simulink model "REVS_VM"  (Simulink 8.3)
settings: Solver=ode3  StartTime=REVS.sim_start_time_secs  StopTime=Inf  FixedStep=REVS.sim_step_time_secs  MaxStep=REVS.sim_step_time_secs
StopFcn:
  | postproc_datalog;
  | postproc_audit;
  | postproc_result;
model workspace (MATLAB code in the model file):
  other statements: REVS_setup_variants
libraries: vehicle_lib x2, ambient_lib x1, driver_lib x1, accessory_lib x1, electric_lib x1, controls_lib x1, engine_lib x1, transmission_lib x1, simulink x1

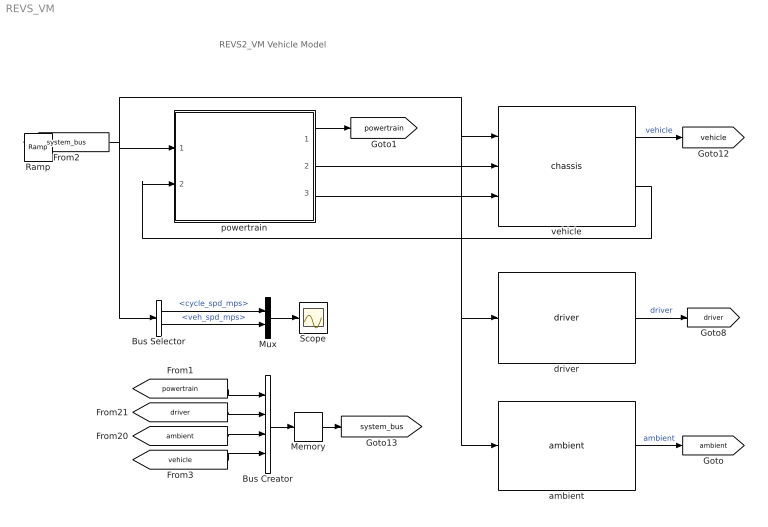
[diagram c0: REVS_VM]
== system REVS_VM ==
  note: REVS2_VM Vehicle Model
  Bus Creator : BusCreator
  Bus Selector : BusSelector  OutputSignals=driver.cycle_spd_mps,vehicle.veh_spd_mps
  Memory : Memory
  Mux : Mux  Inputs=2
  Scope : Scope
  ambient : ambient_lib/ambient
  driver : driver_lib/driver  VariantControl=variants_driver_MT
  powertrain : Subsystem  Variant=on
  vehicle : vehicle_lib/chassis  SystemSampleTime=-1
  Ramp : simulink/Sources/Ramp  IOType=siggen  slope=1  start=0  X0=0
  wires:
  vehicle/1 -> [vehicle]  "vehicle"
  Bus Selector/1 -> Mux/1  "<cycle_spd_mps>"
  Bus Selector/2 -> Mux/2  "<veh_spd_mps>"
  Mux/1 -> Scope/1
  Bus Creator/1 -> Memory/1
  [driver] -> Bus Creator/2
  [ambient] -> Bus Creator/3
  Memory/1 -> [system_bus]
  [system_bus] -> powertrain/1(system_bus), vehicle/1, ambient/1, driver/1, Bus Selector/1
  [powertrain] -> Bus Creator/1
  [vehicle] -> Bus Creator/4
  vehicle/2 -> powertrain/2(veh_spd_mps)
  powertrain/2(force_out_N) -> vehicle/2
  powertrain/3(mass_out_kg) -> vehicle/3
  powertrain/1(bus_out) -> [powertrain]
  ambient/1 -> [ambient]  "ambient"
  driver/1 -> [driver]  "driver"

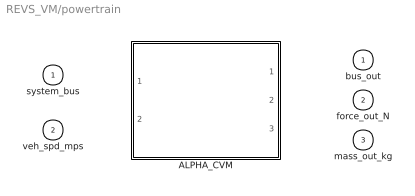
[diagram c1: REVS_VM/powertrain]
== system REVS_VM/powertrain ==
  system_bus : Inport
  veh_spd_mps : Inport  Port=2
  ALPHA_CVM : Subsystem  VariantControl=vehicle_powertrain_type == enum_powertrain_type.conventional && REVS_current_model_type == enum_model_type.ALPHA
  bus_out : Outport
  force_out_N : Outport  Port=2
  mass_out_kg : Outport  Port=3

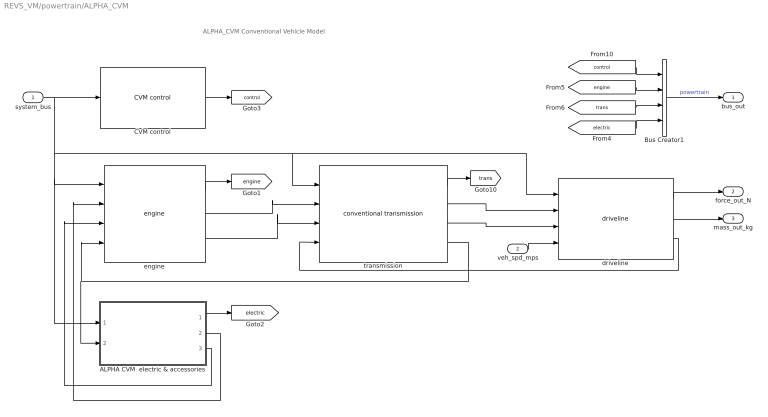
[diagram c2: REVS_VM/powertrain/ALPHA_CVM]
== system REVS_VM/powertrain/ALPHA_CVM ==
  note: ALPHA_CVM Conventional Vehicle Model
  system_bus : Inport
  veh_spd_mps : Inport  Port=2
  ALPHA CVM  electric & accessories : Subsystem  VariantControl=variants_electric_ALPHA
  Bus Creator1 : BusCreator
  CVM control : controls_lib/CVM control
  driveline : vehicle_lib/driveline variants/driveline
  engine : engine_lib/engine  SystemSampleTime=-1
  transmission : transmission_lib/conventional transmission
  bus_out : Outport
  force_out_N : Outport  Port=2
  mass_out_kg : Outport  Port=3
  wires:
  driveline/2 -> mass_out_kg/1
  driveline/1 -> force_out_N/1
  veh_spd_mps/1 -> driveline/4
  system_bus/1 -> ALPHA CVM  electric & accessories/1(system_bus), engine/1, driveline/1, transmission/1, CVM control/1
  [trans] -> Bus Creator1/3
  [engine] -> Bus Creator1/2
  [control] -> Bus Creator1/1
  [electric] -> Bus Creator1/4
  Bus Creator1/1 -> bus_out/1  "powertrain"
  engine/2 -> transmission/2
  transmission/1 -> [trans]
  engine/1 -> [engine]
  transmission/2 -> driveline/2
  ALPHA CVM  electric & accessories/1(bus_out) -> [electric]
  transmission/3 -> driveline/3
  driveline/3 -> transmission/4
  ALPHA CVM  electric & accessories/3(iner_out_kgm2) -> engine/3
  engine/3 -> transmission/3
  transmission/4 -> engine/4, ALPHA CVM  electric & accessories/2(spd_in_radps)
  ALPHA CVM  electric & accessories/2(trq_out_Nm) -> engine/2
  CVM control/1 -> [control]

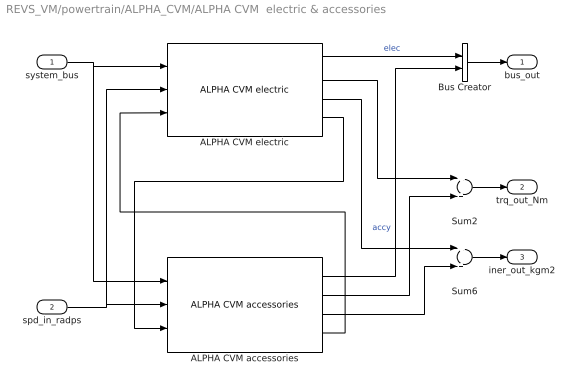
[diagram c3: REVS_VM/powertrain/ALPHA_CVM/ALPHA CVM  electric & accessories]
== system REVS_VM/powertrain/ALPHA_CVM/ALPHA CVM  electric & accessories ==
  system_bus : Inport
  spd_in_radps : Inport  Port=2
  ALPHA CVM accessories : accessory_lib/ALPHA CVM accessories  VariantControl=variants_electric_ALPHA
  ALPHA CVM electric : electric_lib/ALPHA CVM electric  VariantControl=variants_electric_ALPHA
  Bus Creator : BusCreator  Inputs=2
  Sum2 : Sum
  Sum6 : Sum
  bus_out : Outport
  trq_out_Nm : Outport  Port=2
  iner_out_kgm2 : Outport  Port=3
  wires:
  spd_in_radps/1 -> ALPHA CVM accessories/2, ALPHA CVM electric/2
  Bus Creator/1 -> bus_out/1
  system_bus/1 -> ALPHA CVM electric/1, ALPHA CVM accessories/1
  Sum6/1 -> iner_out_kgm2/1
  Sum2/1 -> trq_out_Nm/1
  ALPHA CVM accessories/4 -> ALPHA CVM electric/3
  ALPHA CVM electric/3 -> Sum6/1
  ALPHA CVM electric/1 -> Bus Creator/1  "elec"
  ALPHA CVM accessories/1 -> Bus Creator/2  "accy"
  ALPHA CVM electric/4 -> ALPHA CVM accessories/3
  ALPHA CVM accessories/3 -> Sum6/2
  ALPHA CVM accessories/2 -> Sum2/2
  ALPHA CVM electric/2 -> Sum2/1
